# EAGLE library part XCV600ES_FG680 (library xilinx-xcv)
xcv600es_fg680 edit this description Auto generated by make-symbol-device-package-bsdl.ulp Rev. 26 Source: xcv600es_fg680.bsd
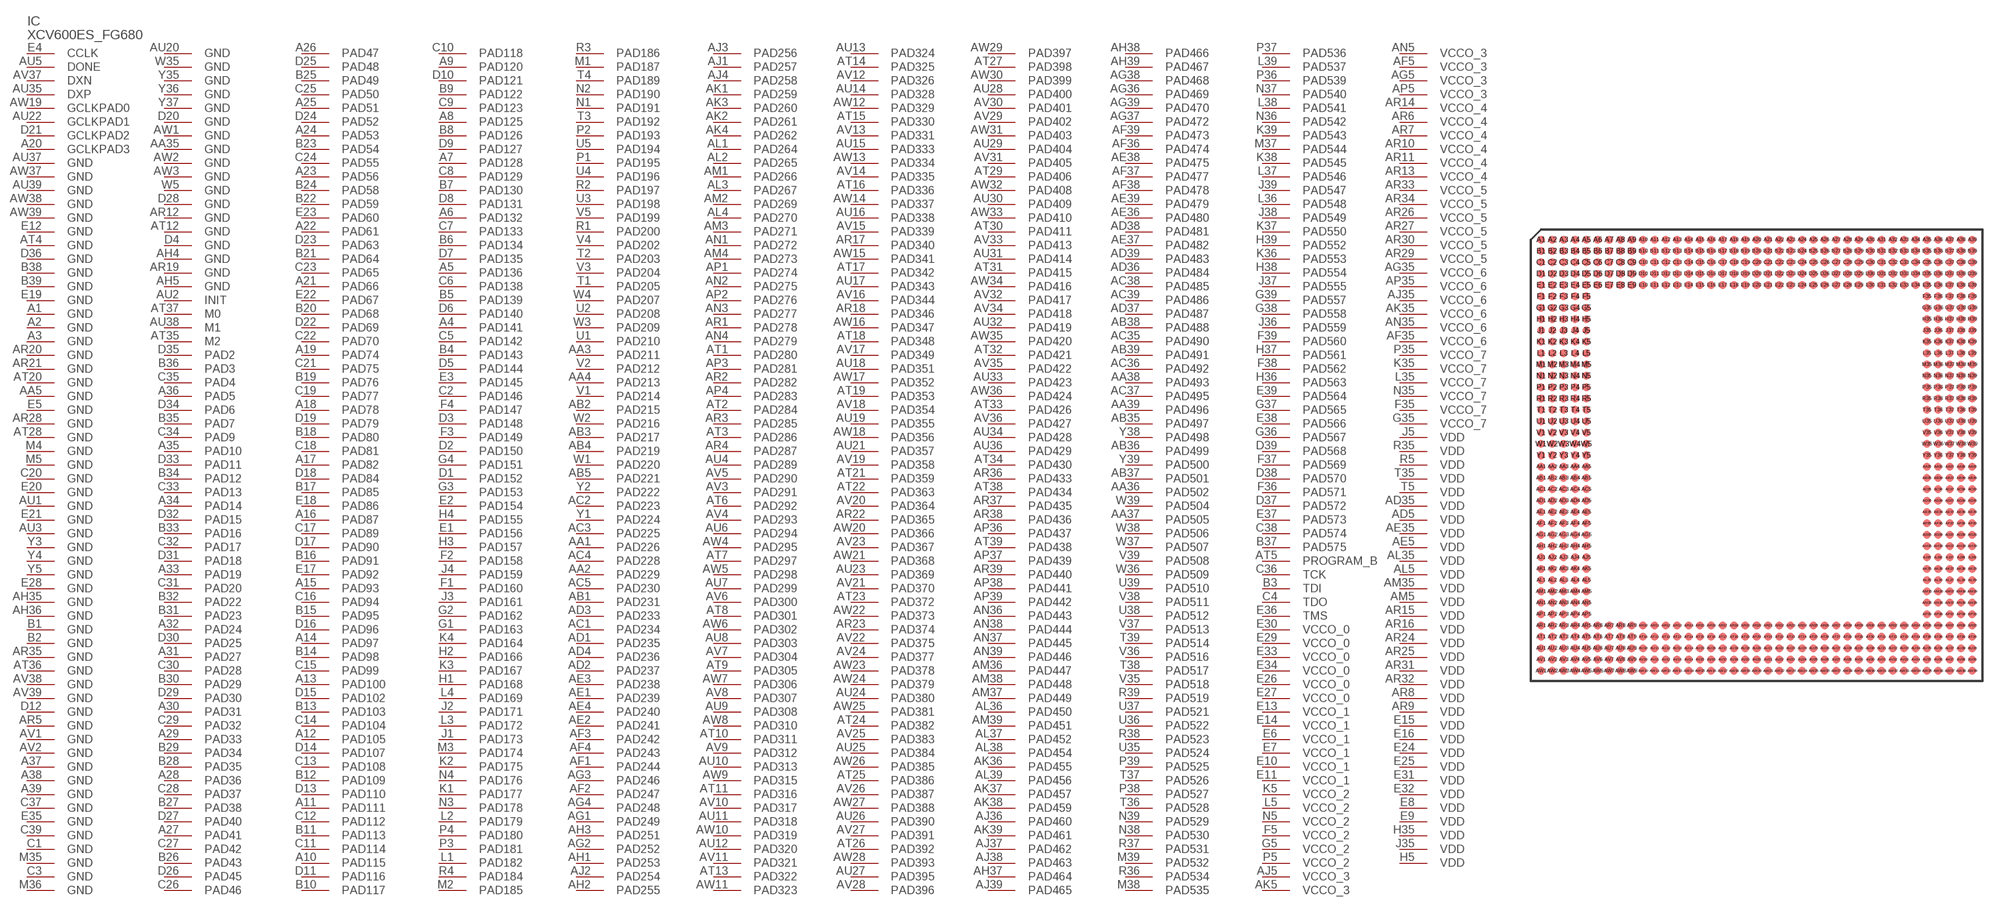
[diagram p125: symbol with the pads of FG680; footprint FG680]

Designator prefix IC

## XCV600ES_FG680 (OC_FARNELL: unknown; OC_NEWARK: unknown)  [FG680]
A1  GND  pwr
A2  GND  pwr
A3  GND  pwr
A4  PAD141
A5  PAD136
A6  PAD132
A7  PAD128
A8  PAD125
A9  PAD120
A10  PAD115
A11  PAD111
A12  PAD105
A13  PAD100
A14  PAD97
A15  PAD93
A16  PAD87
A17  PAD82
A18  PAD78
A19  PAD74
A20  GCLKPAD3  in
A21  PAD66
A22  PAD61
A23  PAD56
A24  PAD53
A25  PAD51
A26  PAD47
A27  PAD41
A28  PAD36
A29  PAD33
A30  PAD31
A31  PAD27
A32  PAD24
A33  PAD19
A34  PAD14
A35  PAD10
A36  PAD5
A37  GND  pwr
A38  GND  pwr
A39  GND  pwr
AA1  PAD226
AA2  PAD229
AA3  PAD211
AA4  PAD213
AA5  GND  pwr
AA35  GND  pwr
AA36  PAD502
AA37  PAD505
AA38  PAD493
AA39  PAD496
AB1  PAD231
AB2  PAD215
AB3  PAD217
AB4  PAD219
AB5  PAD221
AB35  PAD497
AB36  PAD499
AB37  PAD501
AB38  PAD488
AB39  PAD491
AC1  PAD234
AC2  PAD223
AC3  PAD225
AC4  PAD228
AC5  PAD230
AC35  PAD490
AC36  PAD492
AC37  PAD495
AC38  PAD485
AC39  PAD486
AD1  PAD235
AD2  PAD237
AD3  PAD233
AD4  PAD236
AD5  VDD  pwr
AD35  VDD  pwr
AD36  PAD484
AD37  PAD487
AD38  PAD481
AD39  PAD483
AE1  PAD239
AE2  PAD241
AE3  PAD238
AE4  PAD240
AE5  VDD  pwr
AE35  VDD  pwr
AE36  PAD480
AE37  PAD482
AE38  PAD475
AE39  PAD479
AF1  PAD244
AF2  PAD247
AF3  PAD242
AF4  PAD243
AF5  VCCO_3  pwr
AF35  VCCO_6  pwr
AF36  PAD474
AF37  PAD477
AF38  PAD478
AF39  PAD473
AG1  PAD249
AG2  PAD252
AG3  PAD246
AG4  PAD248
AG5  VCCO_3  pwr
AG35  VCCO_6  pwr
AG36  PAD469
AG37  PAD472
AG38  PAD468
AG39  PAD470
AH1  PAD253
AH2  PAD255
AH3  PAD251
AH4  GND  pwr
AH5  GND  pwr
AH35  GND  pwr
AH36  GND  pwr
AH37  PAD464
AH38  PAD466
AH39  PAD467
AJ1  PAD257
AJ2  PAD254
AJ3  PAD256
AJ4  PAD258
AJ5  VCCO_3  pwr
AJ35  VCCO_6  pwr
AJ36  PAD460
AJ37  PAD462
AJ38  PAD463
AJ39  PAD465
AK1  PAD259
AK2  PAD261
AK3  PAD260
AK4  PAD262
AK5  VCCO_3  pwr
AK35  VCCO_6  pwr
AK36  PAD455
AK37  PAD457
AK38  PAD459
AK39  PAD461
AL1  PAD264
AL2  PAD265
AL3  PAD267
AL4  PAD270
AL5  VDD  pwr
AL35  VDD  pwr
AL36  PAD450
AL37  PAD452
AL38  PAD454
AL39  PAD456
AM1  PAD266
AM2  PAD269
AM3  PAD271
AM4  PAD273
AM5  VDD  pwr
AM35  VDD  pwr
AM36  PAD447
AM37  PAD449
AM38  PAD448
AM39  PAD451
AN1  PAD272
AN2  PAD275
AN3  PAD277
AN4  PAD279
AN5  VCCO_3  pwr
AN35  VCCO_6  pwr
AN36  PAD443
AN37  PAD445
AN38  PAD444
AN39  PAD446
AP1  PAD274
AP2  PAD276
AP3  PAD281
AP4  PAD283
AP5  VCCO_3  pwr
AP35  VCCO_6  pwr
AP36  PAD437
AP37  PAD439
AP38  PAD441
AP39  PAD442
AR1  PAD278
AR2  PAD282
AR3  PAD285
AR4  PAD287
AR5  GND  pwr
AR6  VCCO_4  pwr
AR7  VCCO_4  pwr
AR8  VDD  pwr
AR9  VDD  pwr
AR10  VCCO_4  pwr
AR11  VCCO_4  pwr
AR12  GND  pwr
AR13  VCCO_4  pwr
AR14  VCCO_4  pwr
AR15  VDD  pwr
AR16  VDD  pwr
AR17  PAD340
AR18  PAD346
AR19  GND  pwr
AR20  GND  pwr
AR21  GND  pwr
AR22  PAD365
AR23  PAD374
AR24  VDD  pwr
AR25  VDD  pwr
AR26  VCCO_5  pwr
AR27  VCCO_5  pwr
AR28  GND  pwr
AR29  VCCO_5  pwr
AR30  VCCO_5  pwr
AR31  VDD  pwr
AR32  VDD  pwr
AR33  VCCO_5  pwr
AR34  VCCO_5  pwr
AR35  GND  pwr
AR36  PAD433
AR37  PAD435
AR38  PAD436
AR39  PAD440
AT1  PAD280
AT2  PAD284
AT3  PAD286
AT4  GND  pwr
AT5  PROGRAM_B  in
AT6  PAD292
AT7  PAD297
AT8  PAD301
AT9  PAD305
AT10  PAD311
AT11  PAD316
AT12  GND  pwr
AT13  PAD322
AT14  PAD325
AT15  PAD330
AT16  PAD336
AT17  PAD342
AT18  PAD348
AT19  PAD353
AT20  GND  pwr
AT21  PAD359
AT22  PAD363
AT23  PAD372
AT24  PAD382
AT25  PAD386
AT26  PAD392
AT27  PAD398
AT28  GND  pwr
AT29  PAD406
AT30  PAD411
AT31  PAD415
AT32  PAD421
AT33  PAD426
AT34  PAD430
AT35  M2  in
AT36  GND  pwr
AT37  M0  in
AT38  PAD434
AT39  PAD438
AU1  GND  pwr
AU2  INIT
AU3  GND  pwr
AU4  PAD289
AU5  DONE
AU6  PAD294
AU7  PAD299
AU8  PAD303
AU9  PAD308
AU10  PAD313
AU11  PAD318
AU12  PAD320
AU13  PAD324
AU14  PAD328
AU15  PAD333
AU16  PAD338
AU17  PAD343
AU18  PAD351
AU19  PAD355
AU20  GND  pwr
AU21  PAD357
AU22  GCLKPAD1  in
AU23  PAD369
AU24  PAD380
AU25  PAD384
AU26  PAD390
AU27  PAD395
AU28  PAD400
AU29  PAD404
AU30  PAD409
AU31  PAD414
AU32  PAD419
AU33  PAD423
AU34  PAD428
AU35  DXP  pas
AU36  PAD429
AU37  GND  pwr
AU38  M1  in
AU39  GND  pwr
AV1  GND  pwr
AV2  GND  pwr
AV3  PAD291
AV4  PAD293
AV5  PAD290
AV6  PAD300
AV7  PAD304
AV8  PAD307
AV9  PAD312
AV10  PAD317
AV11  PAD321
AV12  PAD326
AV13  PAD331
AV14  PAD335
AV15  PAD339
AV16  PAD344
AV17  PAD349
AV18  PAD354
AV19  PAD358
AV20  PAD364
AV21  PAD370
AV22  PAD375
AV23  PAD367
AV24  PAD377
AV25  PAD383
AV26  PAD387
AV27  PAD391
AV28  PAD396
AV29  PAD402
AV30  PAD401
AV31  PAD405
AV32  PAD417
AV33  PAD413
AV34  PAD418
AV35  PAD422
AV36  PAD427
AV37  DXN  pas
AV38  GND  pwr
AV39  GND  pwr
AW1  GND  pwr
AW2  GND  pwr
AW3  GND  pwr
AW4  PAD295
AW5  PAD298
AW6  PAD302
AW7  PAD306
AW8  PAD310
AW9  PAD315
AW10  PAD319
AW11  PAD323
AW12  PAD329
AW13  PAD334
AW14  PAD337
AW15  PAD341
AW16  PAD347
AW17  PAD352
AW18  PAD356
AW19  GCLKPAD0  in
AW20  PAD366
AW21  PAD368
AW22  PAD373
AW23  PAD378
AW24  PAD379
AW25  PAD381
AW26  PAD385
AW27  PAD388
AW28  PAD393
AW29  PAD397
AW30  PAD399
AW31  PAD403
AW32  PAD408
AW33  PAD410
AW34  PAD416
AW35  PAD420
AW36  PAD424
AW37  GND  pwr
AW38  GND  pwr
AW39  GND  pwr
B1  GND  pwr
B2  GND  pwr
B3  TDI  in
B4  PAD143
B5  PAD139
B6  PAD134
B7  PAD130
B8  PAD126
B9  PAD122
B10  PAD117
B11  PAD113
B12  PAD109
B13  PAD103
B14  PAD98
B15  PAD95
B16  PAD91
B17  PAD85
B18  PAD80
B19  PAD76
B20  PAD68
B21  PAD64
B22  PAD59
B23  PAD54
B24  PAD58
B25  PAD49
B26  PAD43
B27  PAD38
B28  PAD35
B29  PAD34
B30  PAD29
B31  PAD23
B32  PAD22
B33  PAD16
B34  PAD12
B35  PAD7
B36  PAD3
B37  PAD575
B38  GND  pwr
B39  GND  pwr
C1  GND  pwr
C2  PAD146
C3  GND  pwr
C4  TDO  out
C5  PAD142
C6  PAD138
C7  PAD133
C8  PAD129
C9  PAD123
C10  PAD118
C11  PAD114
C12  PAD112
C13  PAD108
C14  PAD104
C15  PAD99
C16  PAD94
C17  PAD89
C18  PAD81
C19  PAD77
C20  GND  pwr
C21  PAD75
C22  PAD70
C23  PAD65
C24  PAD55
C25  PAD50
C26  PAD46
C27  PAD42
C28  PAD37
C29  PAD32
C30  PAD28
C31  PAD20
C32  PAD17
C33  PAD13
C34  PAD9
C35  PAD4
C36  TCK  in
C37  GND  pwr
C38  PAD574
C39  GND  pwr
D1  PAD152
D2  PAD150
D3  PAD148
D4  GND  pwr
D5  PAD144
D6  PAD140
D7  PAD135
D8  PAD131
D9  PAD127
D10  PAD121
D11  PAD116
D12  GND  pwr
D13  PAD110
D14  PAD107
D15  PAD102
D16  PAD96
D17  PAD90
D18  PAD84
D19  PAD79
D20  GND  pwr
D21  GCLKPAD2  in
D22  PAD69
D23  PAD63
D24  PAD52
D25  PAD48
D26  PAD45
D27  PAD40
D28  GND  pwr
D29  PAD30
D30  PAD25
D31  PAD18
D32  PAD15
D33  PAD11
D34  PAD6
D35  PAD2
D36  GND  pwr
D37  PAD572
D38  PAD570
D39  PAD568
E1  PAD156
E2  PAD154
E3  PAD145
E4  CCLK
E5  GND  pwr
E6  VCCO_1  pwr
E7  VCCO_1  pwr
E8  VDD  pwr
E9  VDD  pwr
E10  VCCO_1  pwr
E11  VCCO_1  pwr
E12  GND  pwr
E13  VCCO_1  pwr
E14  VCCO_1  pwr
E15  VDD  pwr
E16  VDD  pwr
E17  PAD92
E18  PAD86
E19  GND  pwr
E20  GND  pwr
E21  GND  pwr
E22  PAD67
E23  PAD60
E24  VDD  pwr
E25  VDD  pwr
E26  VCCO_0  pwr
E27  VCCO_0  pwr
E28  GND  pwr
E29  VCCO_0  pwr
E30  VCCO_0  pwr
E31  VDD  pwr
E32  VDD  pwr
E33  VCCO_0  pwr
E34  VCCO_0  pwr
E35  GND  pwr
E36  TMS  in
E37  PAD573
E38  PAD566
E39  PAD564
F1  PAD160
F2  PAD158
F3  PAD149
F4  PAD147
F5  VCCO_2  pwr
F35  VCCO_7  pwr
F36  PAD571
F37  PAD569
F38  PAD562
F39  PAD560
G1  PAD163
G2  PAD162
G3  PAD153
G4  PAD151
G5  VCCO_2  pwr
G35  VCCO_7  pwr
G36  PAD567
G37  PAD565
G38  PAD558
G39  PAD557
H1  PAD168
H2  PAD166
H3  PAD157
H4  PAD155
H5  VDD  pwr
H35  VDD  pwr
H36  PAD563
H37  PAD561
H38  PAD554
H39  PAD552
J1  PAD173
J2  PAD171
J3  PAD161
J4  PAD159
J5  VDD  pwr
J35  VDD  pwr
J36  PAD559
J37  PAD555
J38  PAD549
J39  PAD547
K1  PAD177
K2  PAD175
K3  PAD167
K4  PAD164
K5  VCCO_2  pwr
K35  VCCO_7  pwr
K36  PAD553
K37  PAD550
K38  PAD545
K39  PAD543
L1  PAD182
L2  PAD179
L3  PAD172
L4  PAD169
L5  VCCO_2  pwr
L35  VCCO_7  pwr
L36  PAD548
L37  PAD546
L38  PAD541
L39  PAD537
M1  PAD187
M2  PAD185
M3  PAD174
M4  GND  pwr
M5  GND  pwr
M35  GND  pwr
M36  GND  pwr
M37  PAD544
M38  PAD535
M39  PAD532
N1  PAD191
N2  PAD190
N3  PAD178
N4  PAD176
N5  VCCO_2  pwr
N35  VCCO_7  pwr
N36  PAD542
N37  PAD540
N38  PAD530
N39  PAD529
P1  PAD195
P2  PAD193
P3  PAD181
P4  PAD180
P5  VCCO_2  pwr
P35  VCCO_7  pwr
P36  PAD539
P37  PAD536
P38  PAD527
P39  PAD525
R1  PAD200
R2  PAD197
R3  PAD186
R4  PAD184
R5  VDD  pwr
R35  VDD  pwr
R36  PAD534
R37  PAD531
R38  PAD523
R39  PAD519
T1  PAD205
T2  PAD203
T3  PAD192
T4  PAD189
T5  VDD  pwr
T35  VDD  pwr
T36  PAD528
T37  PAD526
T38  PAD517
T39  PAD514
U1  PAD210
U2  PAD208
U3  PAD198
U4  PAD196
U5  PAD194
U35  PAD524
U36  PAD522
U37  PAD521
U38  PAD512
U39  PAD510
V1  PAD214
V2  PAD212
V3  PAD204
V4  PAD202
V5  PAD199
V35  PAD518
V36  PAD516
V37  PAD513
V38  PAD511
V39  PAD508
W1  PAD220
W2  PAD216
W3  PAD209
W4  PAD207
W5  GND  pwr
W35  GND  pwr
W36  PAD509
W37  PAD507
W38  PAD506
W39  PAD504
Y1  PAD224
Y2  PAD222
Y3  GND  pwr
Y4  GND  pwr
Y5  GND  pwr
Y35  GND  pwr
Y36  GND  pwr
Y37  GND  pwr
Y38  PAD498
Y39  PAD500

## Footprint FG680 (pad centres in mm)
xcv1000_fg680_1532 edit this description Auto generated by make-symbol-device-package-bsdl.ulp Rev. 26 Source: xcv1000_fg680_1532.bsd
smd 0.7 x 0.7: A1 -19,19; A2 -18,19; A3 -17,19; A4 -16,19; A5 -15,19; A6 -14,19; A7 -13,19; A8 -12,19; A9 -11,19; A10 -10,19; A11 -9,19; A12 -8,19; A13 -7,19; A14 -6,19; A15 -5,19; A16 -4,19; A17 -3,19; A18 -2,19; A19 -1,19; A20 0,19; A21 1,19; A22 2,19; A23 3,19; A24 4,19; A25 5,19; A26 6,19; A27 7,19; A28 8,19; A29 9,19; A30 10,19; A31 11,19; A32 12,19; A33 13,19; A34 14,19; A35 15,19; A36 16,19; A37 17,19; A38 18,19; A39 19,19; AA1 -19,-1; AA2 -18,-1; AA3 -17,-1; AA4 -16,-1; AA5 -15,-1; AA35 15,-1; AA36 16,-1; AA37 17,-1; AA38 18,-1; AA39 19,-1; AB1 -19,-2; AB2 -18,-2; AB3 -17,-2; AB4 -16,-2; AB5 -15,-2; AB35 15,-2; AB36 16,-2; AB37 17,-2; AB38 18,-2; AB39 19,-2; AC1 -19,-3; AC2 -18,-3; AC3 -17,-3; AC4 -16,-3; AC5 -15,-3; AC35 15,-3; AC36 16,-3; AC37 17,-3; AC38 18,-3; AC39 19,-3; AD1 -19,-4; AD2 -18,-4; AD3 -17,-4; AD4 -16,-4; AD5 -15,-4; AD35 15,-4; AD36 16,-4; AD37 17,-4; AD38 18,-4; AD39 19,-4; AE1 -19,-5; AE2 -18,-5; AE3 -17,-5; AE4 -16,-5; AE5 -15,-5; AE35 15,-5; AE36 16,-5; AE37 17,-5; AE38 18,-5; AE39 19,-5; AF1 -19,-6; AF2 -18,-6; AF3 -17,-6; AF4 -16,-6; AF5 -15,-6; AF35 15,-6; AF36 16,-6; AF37 17,-6; AF38 18,-6; AF39 19,-6; AG1 -19,-7; AG2 -18,-7; AG3 -17,-7; AG4 -16,-7; AG5 -15,-7; AG35 15,-7; AG36 16,-7; AG37 17,-7; AG38 18,-7; AG39 19,-7; AH1 -19,-8; AH2 -18,-8; AH3 -17,-8; AH4 -16,-8; AH5 -15,-8; AH35 15,-8; AH36 16,-8; AH37 17,-8; AH38 18,-8; AH39 19,-8; AJ1 -19,-9; AJ2 -18,-9; AJ3 -17,-9; AJ4 -16,-9; AJ5 -15,-9; AJ35 15,-9; AJ36 16,-9; AJ37 17,-9; AJ38 18,-9; AJ39 19,-9; AK1 -19,-10; AK2 -18,-10; AK3 -17,-10; AK4 -16,-10; AK5 -15,-10; AK35 15,-10; AK36 16,-10; AK37 17,-10; AK38 18,-10; AK39 19,-10; AL1 -19,-11; AL2 -18,-11; AL3 -17,-11; AL4 -16,-11; AL5 -15,-11; AL35 15,-11; AL36 16,-11; AL37 17,-11; AL38 18,-11; AL39 19,-11; AM1 -19,-12; AM2 -18,-12; AM3 -17,-12; AM4 -16,-12; AM5 -15,-12; AM35 15,-12; AM36 16,-12; AM37 17,-12; AM38 18,-12; AM39 19,-12; AN1 -19,-13; AN2 -18,-13; AN3 -17,-13; AN4 -16,-13; AN5 -15,-13; AN35 15,-13; AN36 16,-13; AN37 17,-13; AN38 18,-13; AN39 19,-13; AP1 -19,-14; AP2 -18,-14; AP3 -17,-14; AP4 -16,-14; AP5 -15,-14; AP35 15,-14; AP36 16,-14; AP37 17,-14; AP38 18,-14; AP39 19,-14; AR1 -19,-15; AR2 -18,-15; AR3 -17,-15; AR4 -16,-15; AR5 -15,-15; AR6 -14,-15; AR7 -13,-15; AR8 -12,-15; AR9 -11,-15; AR10 -10,-15; AR11 -9,-15; AR12 -8,-15; AR13 -7,-15; AR14 -6,-15; AR15 -5,-15; AR16 -4,-15; AR17 -3,-15; AR18 -2,-15; AR19 -1,-15; AR20 0,-15; AR21 1,-15; AR22 2,-15; AR23 3,-15; AR24 4,-15; AR25 5,-15; AR26 6,-15; AR27 7,-15; AR28 8,-15; AR29 9,-15; AR30 10,-15; AR31 11,-15; AR32 12,-15; AR33 13,-15; AR34 14,-15; AR35 15,-15; AR36 16,-15; AR37 17,-15; AR38 18,-15; AR39 19,-15; AT1 -19,-16; AT2 -18,-16; AT3 -17,-16; AT4 -16,-16; AT5 -15,-16; AT6 -14,-16; AT7 -13,-16; AT8 -12,-16; AT9 -11,-16; AT10 -10,-16; AT11 -9,-16; AT12 -8,-16; AT13 -7,-16; AT14 -6,-16; AT15 -5,-16; AT16 -4,-16; AT17 -3,-16; AT18 -2,-16; AT19 -1,-16; AT20 0,-16; AT21 1,-16; AT22 2,-16; AT23 3,-16; AT24 4,-16; AT25 5,-16; AT26 6,-16; AT27 7,-16; AT28 8,-16; AT29 9,-16; AT30 10,-16; AT31 11,-16; AT32 12,-16; AT33 13,-16; AT34 14,-16; AT35 15,-16; AT36 16,-16; AT37 17,-16; AT38 18,-16; AT39 19,-16; AU1 -19,-17; AU2 -18,-17; AU3 -17,-17; AU4 -16,-17; AU5 -15,-17; AU6 -14,-17; AU7 -13,-17; AU8 -12,-17; AU9 -11,-17; AU10 -10,-17; AU11 -9,-17; AU12 -8,-17; AU13 -7,-17; AU14 -6,-17; AU15 -5,-17; AU16 -4,-17; AU17 -3,-17; AU18 -2,-17; AU19 -1,-17; AU20 0,-17; AU21 1,-17; AU22 2,-17; AU23 3,-17; AU24 4,-17; AU25 5,-17; AU26 6,-17; AU27 7,-17; AU28 8,-17; AU29 9,-17; AU30 10,-17; AU31 11,-17; AU32 12,-17; AU33 13,-17; AU34 14,-17; AU35 15,-17; AU36 16,-17; AU37 17,-17; AU38 18,-17; AU39 19,-17; AV1 -19,-18; AV2 -18,-18; AV3 -17,-18; AV4 -16,-18; AV5 -15,-18; AV6 -14,-18; AV7 -13,-18; AV8 -12,-18; AV9 -11,-18; AV10 -10,-18; AV11 -9,-18; AV12 -8,-18; AV13 -7,-18; AV14 -6,-18; AV15 -5,-18; AV16 -4,-18; AV17 -3,-18; AV18 -2,-18; AV19 -1,-18; AV20 0,-18; AV21 1,-18; AV22 2,-18; AV23 3,-18; AV24 4,-18; AV25 5,-18; AV26 6,-18; AV27 7,-18; AV28 8,-18; AV29 9,-18; AV30 10,-18; AV31 11,-18; AV32 12,-18; AV33 13,-18; AV34 14,-18; AV35 15,-18; AV36 16,-18; AV37 17,-18; AV38 18,-18; AV39 19,-18; AW1 -19,-19; AW2 -18,-19; AW3 -17,-19; AW4 -16,-19; AW5 -15,-19; AW6 -14,-19; AW7 -13,-19; AW8 -12,-19; AW9 -11,-19; AW10 -10,-19; AW11 -9,-19; AW12 -8,-19; AW13 -7,-19; AW14 -6,-19; AW15 -5,-19; AW16 -4,-19; AW17 -3,-19; AW18 -2,-19; AW19 -1,-19; AW20 0,-19; AW21 1,-19; AW22 2,-19; AW23 3,-19; AW24 4,-19; AW25 5,-19; AW26 6,-19; AW27 7,-19; AW28 8,-19; AW29 9,-19; AW30 10,-19; AW31 11,-19; AW32 12,-19; AW33 13,-19; AW34 14,-19; AW35 15,-19; AW36 16,-19; AW37 17,-19; AW38 18,-19; AW39 19,-19; B1 -19,18; B2 -18,18; B3 -17,18; B4 -16,18; B5 -15,18; B6 -14,18; B7 -13,18; B8 -12,18; B9 -11,18; B10 -10,18; B11 -9,18; B12 -8,18; B13 -7,18; B14 -6,18; B15 -5,18; B16 -4,18; B17 -3,18; B18 -2,18; B19 -1,18; B20 0,18; B21 1,18; B22 2,18; B23 3,18; B24 4,18; B25 5,18; B26 6,18; B27 7,18; B28 8,18; B29 9,18; B30 10,18; B31 11,18; B32 12,18; B33 13,18; B34 14,18; B35 15,18; B36 16,18; B37 17,18; B38 18,18; B39 19,18; C1 -19,17; C2 -18,17; C3 -17,17; C4 -16,17; C5 -15,17; C6 -14,17; C7 -13,17; C8 -12,17; C9 -11,17; C10 -10,17; C11 -9,17; C12 -8,17; C13 -7,17; C14 -6,17; C15 -5,17; C16 -4,17; C17 -3,17; C18 -2,17; C19 -1,17; C20 0,17; C21 1,17; C22 2,17; C23 3,17; C24 4,17; C25 5,17; C26 6,17; C27 7,17; C28 8,17; C29 9,17; C30 10,17; C31 11,17; C32 12,17; C33 13,17; C34 14,17; C35 15,17; C36 16,17; C37 17,17; C38 18,17; C39 19,17; D1 -19,16; D2 -18,16; D3 -17,16; D4 -16,16; D5 -15,16; D6 -14,16; D7 -13,16; D8 -12,16; D9 -11,16; D10 -10,16; D11 -9,16; D12 -8,16; D13 -7,16; D14 -6,16; D15 -5,16; D16 -4,16; D17 -3,16; D18 -2,16; D19 -1,16; D20 0,16; D21 1,16; D22 2,16; D23 3,16; D24 4,16; D25 5,16; D26 6,16; D27 7,16; D28 8,16; D29 9,16; D30 10,16; D31 11,16; D32 12,16; D33 13,16; D34 14,16; D35 15,16; D36 16,16; D37 17,16; D38 18,16; D39 19,16; E1 -19,15; E2 -18,15; E3 -17,15; E4 -16,15; E5 -15,15; E6 -14,15; E7 -13,15; E8 -12,15; E9 -11,15; E10 -10,15; E11 -9,15; E12 -8,15; E13 -7,15; E14 -6,15; E15 -5,15; E16 -4,15; E17 -3,15; E18 -2,15; E19 -1,15; E20 0,15; E21 1,15; E22 2,15; E23 3,15; E24 4,15; E25 5,15; E26 6,15; E27 7,15; E28 8,15; E29 9,15; E30 10,15; E31 11,15; E32 12,15; E33 13,15; E34 14,15; E35 15,15; E36 16,15; E37 17,15; E38 18,15; E39 19,15; F1 -19,14; F2 -18,14; F3 -17,14; F4 -16,14; F5 -15,14; F35 15,14; F36 16,14; F37 17,14; F38 18,14; F39 19,14; G1 -19,13; G2 -18,13; G3 -17,13; G4 -16,13; G5 -15,13; G35 15,13; G36 16,13; G37 17,13; G38 18,13; G39 19,13; H1 -19,12; H2 -18,12; H3 -17,12; H4 -16,12; H5 -15,12; H35 15,12; H36 16,12; H37 17,12; H38 18,12; H39 19,12; J1 -19,11; J2 -18,11; J3 -17,11; J4 -16,11; J5 -15,11; J35 15,11; J36 16,11; J37 17,11; J38 18,11; J39 19,11; K1 -19,10; K2 -18,10; K3 -17,10; K4 -16,10; K5 -15,10; K35 15,10; K36 16,10; K37 17,10; K38 18,10; K39 19,10; L1 -19,9; L2 -18,9; L3 -17,9; L4 -16,9; L5 -15,9; L35 15,9; L36 16,9; L37 17,9; L38 18,9; L39 19,9; M1 -19,8; M2 -18,8; M3 -17,8; M4 -16,8; M5 -15,8; M35 15,8; M36 16,8; M37 17,8; M38 18,8; M39 19,8; N1 -19,7; N2 -18,7; N3 -17,7; N4 -16,7; N5 -15,7; N35 15,7; N36 16,7; N37 17,7; N38 18,7; N39 19,7; P1 -19,6; P2 -18,6; P3 -17,6; P4 -16,6; P5 -15,6; P35 15,6; P36 16,6; P37 17,6; P38 18,6; P39 19,6; R1 -19,5; R2 -18,5; R3 -17,5; R4 -16,5; R5 -15,5; R35 15,5; R36 16,5; R37 17,5; R38 18,5; R39 19,5; T1 -19,4; T2 -18,4; T3 -17,4; T4 -16,4; T5 -15,4; T35 15,4; T36 16,4; T37 17,4; T38 18,4; T39 19,4; U1 -19,3; U2 -18,3; U3 -17,3; U4 -16,3; U5 -15,3; U35 15,3; U36 16,3; U37 17,3; U38 18,3; U39 19,3; V1 -19,2; V2 -18,2; V3 -17,2; V4 -16,2; V5 -15,2; V35 15,2; V36 16,2; V37 17,2; V38 18,2; V39 19,2; W1 -19,1; W2 -18,1; W3 -17,1; W4 -16,1; W5 -15,1; W35 15,1; W36 16,1; W37 17,1; W38 18,1; W39 19,1; Y1 -19,0; Y2 -18,0; Y3 -17,0; Y4 -16,0; Y5 -15,0; Y35 15,0; Y36 16,0; Y37 17,0; Y38 18,0; Y39 19,0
